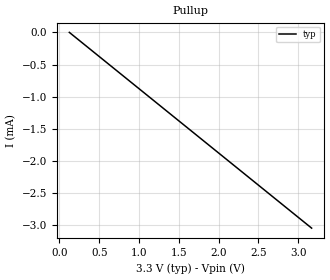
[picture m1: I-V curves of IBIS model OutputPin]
[IBIS Ver]   2.1
[File Name]   bug33.ibs
[File Rev]   0.1
[Component]   TEST
[Manufacturer]   Test File
[Package]
| variable   typ   min   max
R_pkg   0.0m   NA   NA
L_pkg   0.0nH   NA   NA
C_pkg   0.0pF   NA   NA
[Pin]   signal_name   model_name
1   One_Pin   OutputPin
| Models and submodels in the file (1): OutputPin (Output)
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[Model]   OutputPin
Model_type   Output
Vmeas = 1.2V
Cref = 5pF
Rref = 50
Vref = 1.2
| variable   typ   min   max
C_comp   6.763pF   NA   NA
[Temperature Range]   25.0   NA   NA
[Voltage range]   3.3V   NA   NA
[Pullup]
|Voltage   I(typ)   I(min)   I(max)
*3.3   -3.0580E-03   NA   NA
123.5mV   4.429nA    NA         NA
3.168V    -3.045mA   NA         NA
[Ramp]
|   typ   min   max
dV/dt_r   1.0/1.0n   NA   NA
dV/dt_f   1.0/1.0n   NA   NA
